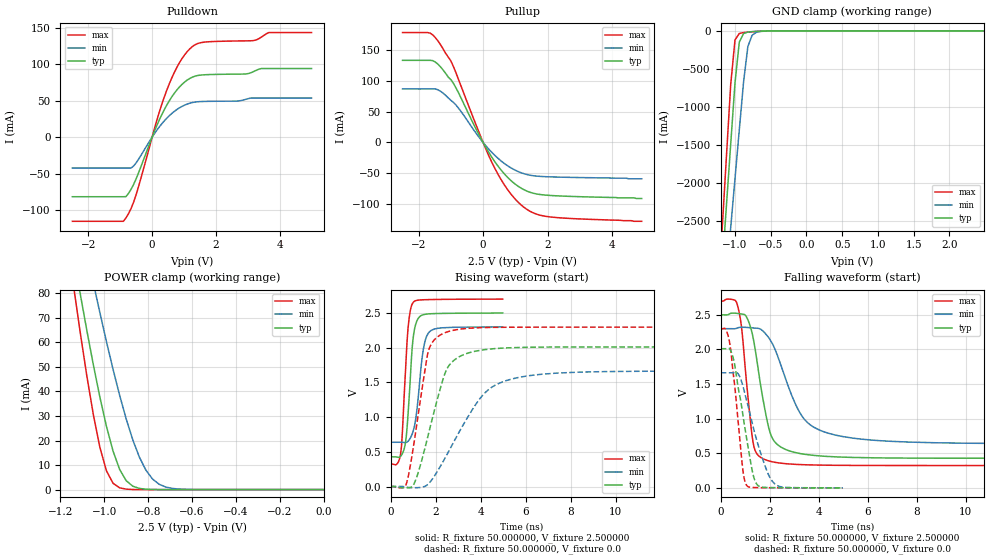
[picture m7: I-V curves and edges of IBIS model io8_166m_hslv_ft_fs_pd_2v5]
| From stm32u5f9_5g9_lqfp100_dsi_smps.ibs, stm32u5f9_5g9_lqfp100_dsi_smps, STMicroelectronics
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|   Model io8_166m_hslv_ft_fs_pd_2v5
[Model]  io8_166m_hslv_ft_fs_pd_2v5
Model_type I/O
Polarity   Non-Inverting
Enable   Active-Low
Vinl =   0.750000V
Vinh =   1.750000V
Vmeas =  1.250000V
Cref =   50.000000pF
Rref =   100.000000M
Vref =   0.0V
C_comp   3.458600pF   3.458000pF   3.495600pF
[Temperature Range]   25.000000   0.140000k   -40.000000
[Pullup Reference]   2.500000V   2.300000V   2.700000V
[Pulldown Reference]   0.0V   0.0V   0.0V
[POWER Clamp Reference]   2.500000V   2.300000V   2.700000V
[GND Clamp Reference]   0.0V   0.0V   0.0V
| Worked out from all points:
|   slope of the pulldown table from 0 to 0.375 V, typ, clamps not added: 10.1 ohm
|   slope of the pullup table from 0 to 0.375 V, typ, clamps not added: 11.7 ohm
|   GND clamp passes 1 mA (typ) near -0.50 V on its own axis
|   POWER clamp passes 1 mA (typ) near -0.86 V on its own axis
|   rising waveform, R_fixture 50.000000, V_fixture 2.500000: 20-80 % time 255ps typ, 337ps min, 236ps max; typ from 0.427 V to 2.5 V
|   rising waveform, R_fixture 50.000000, V_fixture 0.0: 20-80 % time 989ps typ, 1.85ns min, 648ps max; typ from 0 V to 2.01 V
|   falling waveform, R_fixture 50.000000, V_fixture 2.500000: 20-80 % time 613ps typ, 1.21ns min, 386ps max; typ from 2.5 V to 0.427 V
|   falling waveform, R_fixture 50.000000, V_fixture 0.0: 20-80 % time 561ps typ, 786ps min, 389ps max; typ from 2.01 V to 0 V
[Pulldown]
|Voltage   I(typ)   I(min)   I(max)
-2.5V     -81.61mA   -42.31mA   -115.3mA
-900mV    -81.61mA   -42.31mA   -115.3mA
-820mV    -81.43mA   -42.31mA   -110.6mA
-500mV    -56.95mA   -35.08mA   -78.57mA
140mV     15.18mA    9.02mA     22.02mA
460mV     44mA       25.98mA    64.38mA
860mV     68.91mA    40.27mA    102.2mA
1.26V     82.21mA    47.42mA    124mA
1.66V     85.54mA    49mA       130.3mA
3.18V     89.84mA    53.64mA    132.3mA
3.66V     94.01mA    53.64mA    143.3mA
5V        94.01mA    53.64mA    143.3mA
[Pullup]
|Voltage   I(typ)   I(min)   I(max)
-2.5V     133.3mA    86.84mA    178.4mA
-1.64V    133.3mA    86.84mA    177.4mA
-1.4V     127mA      85.44mA    164.7mA
-1V       102mA      68.42mA    132.3mA
-920mV    95.91mA    64.95mA    123.1mA
-120mV    11.82mA    8.046mA    15.6mA
360mV     -30.97mA   -20.78mA   -41.56mA
760mV     -56.64mA   -37.85mA   -76.55mA
1.24V     -75.99mA   -50.28mA   -104.1mA
1.64V     -83.42mA   -54.54mA   -116.1mA
2.04V     -85.88mA   -55.77mA   -120.7mA
4.92V     -91mA      -59mA      -128mA
[GND_clamp]
|Voltage   I(typ)   I(min)   I(max)
-2.5V     -9.641A    -9.693A    -9.352A
-1.18V    -3.114A    -3.874A    -2.614A
-1.12V    -2.301A    -3.23A     -1.656A
-1.06V    -1.489A    -2.587A    -706.2mA
-1V       -685.8mA   -1.945A    -119.3mA
-940mV    -149.8mA   -1.304A    -34.74mA
-880mV    -35.55mA   -672.6mA   -23.08mA
-820mV    -16.21mA   -206.4mA   -17.29mA
-760mV    -10.59mA   -57.56mA   -12.42mA
-700mV    -7.163mA   -18.75mA   -8.254mA
-400mV    -112.4uA   -385.2uA   -53.47uA
2.48V     63.1uA     48.03uA    77.39uA
[POWER_clamp]
|Voltage   I(typ)   I(min)   I(max)
-2.49V    881mA      773.1mA    1.07A
-1.14V    95.25mA    122.7mA    82.82mA
-1.11V    79.9mA     109.7mA    64.14mA
-1.05V    50.87mA    84.26mA    30.57mA
-1.02V    37.63mA    72.04mA    17.17mA
-990mV    25.71mA    60.25mA    7.621mA
-930mV    8.217mA    38.43mA    713.9uA
-900mV    3.624mA    28.77mA    182.8uA
-840mV    490.7uA    13.24mA    11.35uA
-780mV    56.55uA    4.324mA    699nA
-660mV    716.7nA    226uA      9.784nA
0V        0A         19.53nA    0A
[Ramp]
| variable   typ   min   max
dV/dt_r  1.20630/0.98810n   0.99744/1.84649n   1.37748/0.64660n
dV/dt_f  1.24322/0.61158n   0.99725/1.21040n   1.42605/0.38517n
R_load = 50.000000
[Rising Waveform]
R_fixture= 50.000000
V_fixture= 2.500000
V_fixture_min= 2.300000
V_fixture_max= 2.700000
|time   V(typ)   V(min)   V(max)
0s        427.4mV    637.3mV    322.7mV
450.5ps   437.1mV    637.3mV    479.4mV
520.5ps   472.1mV    636.6mV    760mV
640.6ps   592.4mV    633mV      1.532V
790.8ps   1.11V      656.6mV    2.326V
991ps     2.101V     784.5mV    2.646V
1.161ns   2.378V     1.081V     2.681V
1.451ns   2.475V     1.966V     2.69V
1.732ns   2.488V     2.23V      2.693V
4.985ns   2.499V     2.299V     2.7V
[Rising Waveform]
R_fixture= 50.000000
V_fixture= 0.0
V_fixture_min= 0.0
V_fixture_max= 0.0
|time   V(typ)   V(min)   V(max)
0s        -56.37uV   -13.69uV   871.7nV
680.7ps   -19.35mV   -7.041mV   20.91mV
1.041ns   37.96mV    -17.08mV   626.4mV
1.682ns   753.4mV    38.25mV    1.952V
1.962ns   1.113V     157.1mV    2.12V
2.442ns   1.65V      423.1mV    2.219V
3.003ns   1.86V      758mV      2.263V
4.124ns   1.969V     1.326V     2.289V
5.646ns   2.002V     1.568V     2.295V
19.94ns   2.011V     1.663V     2.296V
[Falling Waveform]
R_fixture= 50.000000
V_fixture= 2.500000
V_fixture_min= 2.300000
V_fixture_max= 2.700000
|time   V(typ)   V(min)   V(max)
0s        2.499V     2.299V     2.7V
680.7ps   2.52V      2.31V      2.643V
840.8ps   2.511V     2.32V      2.347V
1.081ns   2.449V     2.317V     1.425V
1.361ns   2.095V     2.309V     587.6mV
1.882ns   990.8mV    2.204V     398.3mV
2.282ns   635.4mV    1.942V     365.1mV
3.323ns   490.7mV    1.033V     335.3mV
4.645ns   448.6mV    765.5mV    326mV
19.94ns   427.4mV    637.3mV    322.7mV
[Falling Waveform]
R_fixture= 50.000000
V_fixture= 0.0
V_fixture_min= 0.0
V_fixture_max= 0.0
|time   V(typ)   V(min)   V(max)
0s        2.011V     1.663V     2.296V
200.2ps   2.01V      1.663V     2.291V
370.4ps   2.005V     1.663V     2.085V
560.6ps   1.796V     1.666V     1.509V
900.9ps   1.065V     1.478V     268.5mV
1.071ns   684.4mV    1.243V     31.06mV
1.291ns   240mV      928.5mV    6.157mV
1.451ns   64.55mV    711mV      4.051mV
2.182ns   2.949mV    65.11mV    1.529mV
4.985ns   -56.37uV   -13.69uV   871.7nV
